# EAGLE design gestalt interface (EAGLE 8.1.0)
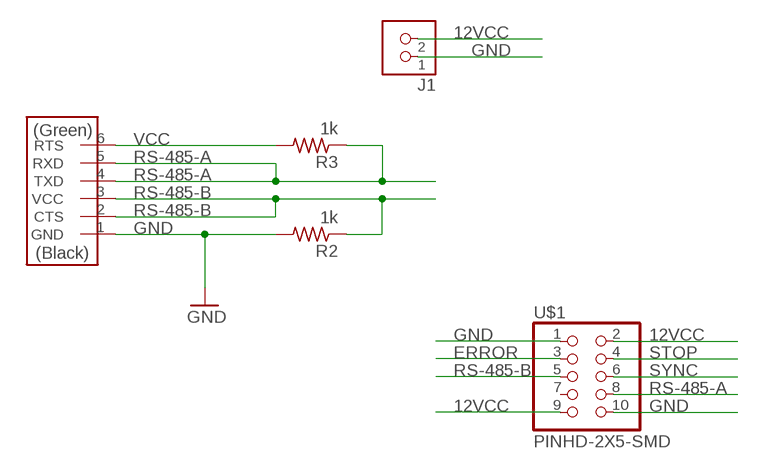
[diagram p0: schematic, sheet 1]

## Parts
J1  TERM-1X02-FABLAB  [ED555DS-2DS]
R2  1k  RES-US1206FAB  [R1206FAB]
R3  1k  RES-US1206FAB  [R1206FAB]
U$1  PINHD-2X5-SMD  [2X05SMD]
U$2  FTDI-SMD-HEADER  [1X06SMD]

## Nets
12VCC: J1.2 U$1.2 U$1.9
ERROR: U$1.3
GND: J1.1 R2.2 U$1.1 U$1.10 U$2.1(GND)
RS-485-A: R3.1 U$1.8 U$2.4(TXD) U$2.5(RXD)
RS-485-B: R2.1 U$1.5 U$2.2(CTS) U$2.3(VCC)
STOP: U$1.4
SYNC: U$1.6
VCC: R3.2 U$2.6(RTS)
Unconnected: U$1.7

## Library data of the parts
J1 = fab:TERM-1X02: 3.5mm terminal block, 2 positions ED555-2DS as found in the fablab inventory.
R2 R3 = fab:RES-US: Resistor (US Symbol)
U$1 = fab:PINHD-2X5-SMD
U$2 = fab:FTDI-SMD-HEADER

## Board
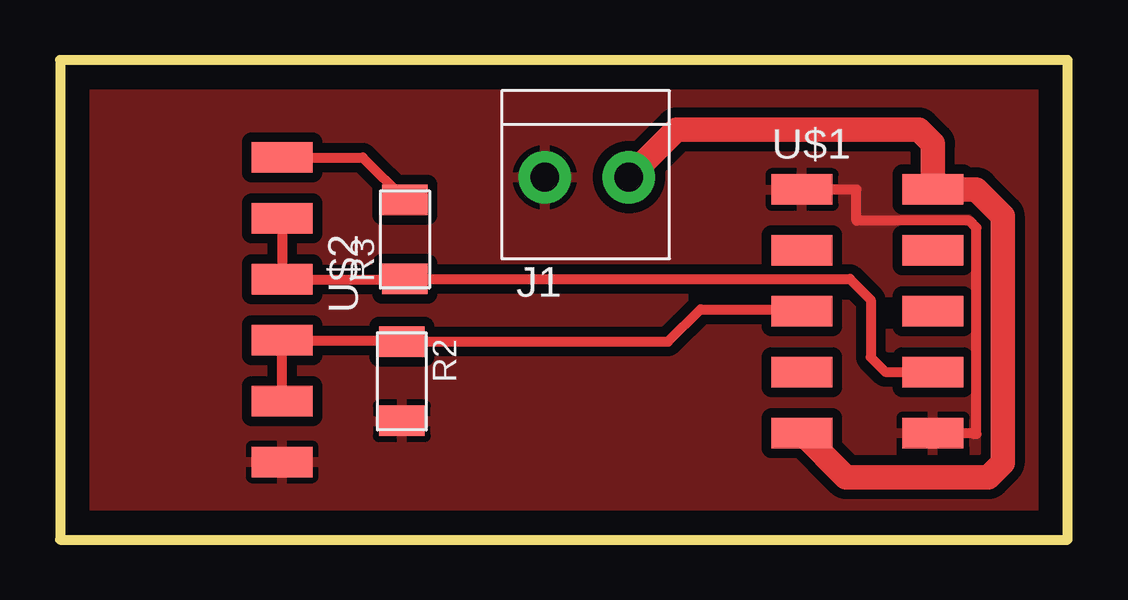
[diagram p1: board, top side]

Size 42 x 20 mm. Coordinates in mm from the lower left corner, seen from the top.
Outline: 0,0 42,0 42,20 0,20 0,0
Copper layers (1*16): Top 0.035mm / dielectric 1.5mm / Bottom 0.035mm
Design rules "default": minimum track width 10mil, minimum drill 24mil, track to track 8mil, track to pad 8mil, pad to pad 8mil, via to via 8mil, smd to smd 8mil, copper to edge 40mil, drill to drill 8mil, minimum pad ring 10mil, minimum via ring 8mil, stop-mask expansion 4mil, vias tented up to drill 0mil, thermal gap 10mil

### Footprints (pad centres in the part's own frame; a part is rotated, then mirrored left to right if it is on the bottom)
ED555DS-2DS = drill 1.2 pad 2.184: 1 1.8,0; 2 -1.7,0
R1206FAB = smd 1.27 x 1.905: 1 -1.651,0; 2 1.651,0
2X05SMD = smd 2.54 x 1.27: 1 -2.54,2.54; 2 2.92,2.54; 3 -2.54,0; 4 2.92,0; 5 -2.54,-2.54; 6 2.92,-2.54; 7 -2.54,-5.08; 8 2.92,-5.08; 9 -2.54,-7.62; 10 2.92,-7.62
1X06SMD = smd 2.54 x 1.27: 1 0,6.35; 2 0,3.81; 3 0,1.27; 4 0,-1.27; 5 0,-3.81; 6 0,-6.35

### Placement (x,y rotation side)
J1  22.01,15.11 180 top
R2  14.25,6.6 270 top
R3  14.38,12.52 90 top
U$1  33.47,12.06 0 top
U$2  9.26,9.58 180 top

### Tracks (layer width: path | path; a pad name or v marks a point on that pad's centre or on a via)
12VCC
  Top 1.016: U$1.9 32.77,2.6 38.7,2.6 39.3,3.2 39.3,13.5 38.2,14.6 U$1.2 36.39,16.51 35.8,17.1 25.7,17.1 J1.2
GND
  Top 0.406: U$1.10 38.1,4.44 38.1,4.4 38.2,4.4 38.2,13 37.9,13.3 33.2,13.3 33.2,14.6 U$1.1
  pour Top (isolate 0.406): 0,0 41,0 41,19 0,19
RS-485-A
  Top 0.406: U$2.5 U$2.4 14.36,10.85 R3.1 32.93,10.87 33.8,10 33.8,7.6 34.4,7 36.37,7 U$1.8
RS-485-B
  Top 0.406: U$2.2 U$2.3 14.19,8.31 R2.1 25.35,8.25 26.7,9.6 30.85,9.6 U$1.5
VCC
  Top 0.406: U$2.6 12.62,15.93 R3.2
